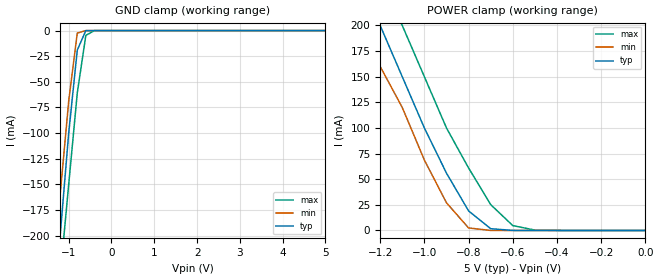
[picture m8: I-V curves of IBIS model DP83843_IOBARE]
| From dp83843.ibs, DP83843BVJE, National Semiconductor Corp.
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|   Model DP83843_IOBARE
|Note: Analog inputs modeled as IOBARE pad inorder to provide DC
|   PWR/GND_clamp characteristics.  Vinl/Vinh do not necessarily
|   apply, see datasheet.
[Model]   DP83843_IOBARE
Model_type   Input
Vinl =   0.80V
Vinh =   2.00V
Vmeas =   1.50V
C_comp   5.83pF   5.83pF   5.83pF
[Temperature Range]   50.00   -15.00   0.15k
[Voltage Range]   5.00V   4.50V   5.50V
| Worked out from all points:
|   GND clamp passes 1 mA (typ) near -0.61 V on its own axis
|   POWER clamp passes 1 mA (typ) near -0.66 V on its own axis
[GND_clamp]
| voltage   I(typ)   I(min)   I(max)
-5V       -2.16A     -2.13A     -2.2A
-1.4V     -290mA     -260mA     -340mA
-1.2V     -200mA     -160mA     -240mA
-1V       -100mA     -68.72mA   -150mA
-800mV    -19.09mA   -2.46mA    -60.97mA
-600mV    -53.29uA   -380nA     -4.74mA
-400mV    -40.77nA   -52.67pA   -25.25uA
5V        5.02pA     4.24nA     4.5pA
[POWER_clamp]
| voltage   I(typ)   I(min)   I(max)
-5V       2.16A      2.13A      2.2A
-1.3V     240mA      210mA      290mA
-1.2V     200mA      160mA      240mA
-1.1V     150mA      120mA      200mA
-1V       100mA      68.72mA    150mA
-900mV    55.95mA    27.02mA    100mA
-800mV    19.09mA    2.46mA     60.97mA
-700mV    1.72mA     33.83uA    25.26mA
-600mV    53.29uA    380nA      4.74mA
-500mV    1.48uA     4.24nA     380uA
0V        5.02pA     4.5pA      440pA
